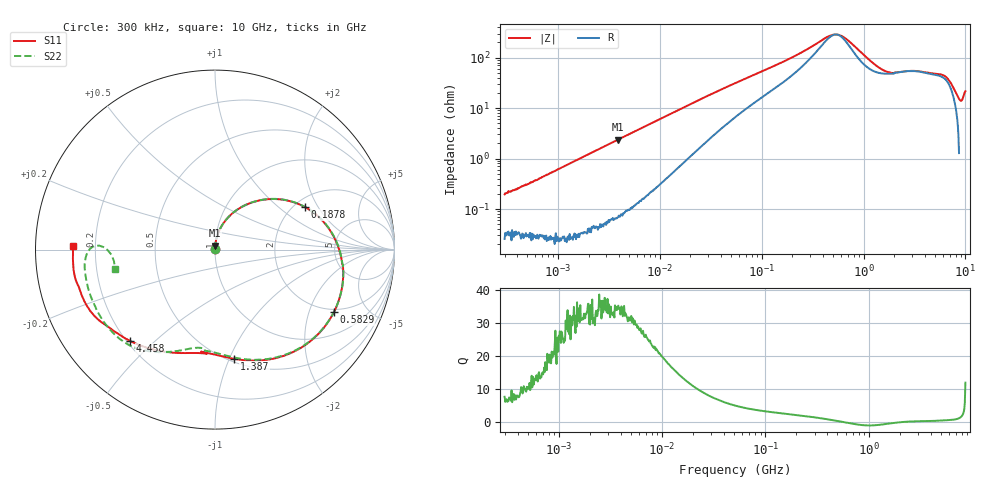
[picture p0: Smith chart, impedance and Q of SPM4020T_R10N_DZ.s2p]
! S-Parameter Data Generated by TDK Corporation
! Copyright(C) 2024 TDK Corporation.
! All Rights Reserved.
! TDK P/N: SPM4020T-R10N-DZ (SMD / SMT Inductor (Coil))
! Property: L=100nH at 100kHz
! Size(LxWxT): 4.3x4.1x2mm
! Model Type: s2p (Touchstone File Format Version 1.0)
! Frequency: DC=Yes Start=0.3MHz Stop=10000MHz 802points Log-sweep
! Model Generated on May 28, 2024
! Terms and conditions regarding TDK Simulation Models:
! 1)This simulation model is being provided solely for informational
!  purposes. Please refer to the specifications of the products in
!  terms of detailed characteristics of such products.
! 2)In no event shall TDK Corporation of any of its subsidiaries be
!  liable for any loss or damage arising, directly or indirectly,
!  from any information contained in this simulation model, including,
!  but not limited to loss or damages arising from any inaccuracies,
!  omissions or errors in connection with such information.
! 3)Any and all copyrights on this simulation model are owned by
!  TDK Corporation.  Duplication or redistribution of this simulation
!  model without prior written permission from TDK Corporation
!  is prohibited.
! 4)This simulation model is subject to any modification or change
!  without any prior notice.
! 5)Neither TDK Corporation nor any of its subsidiaries shall make any
!  warranty, express or implied, including but not limited to the
!  correctness, implied warranties of merchantability and fitness for
!  a particular purpose with respect to this simulation models.
! 6)The use of this simulation model shall be deemed to have consented
!  to the terms and conditions hereof.
! Port Assignments:
!  1 ---@@@--- 2
! Applicable Conditions:
!  Temperature = 25 degC
!  DC Bias Current = 0 A
!  Small Signal Operation
# Hz S MA R 50
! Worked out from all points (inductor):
!   801 points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, 300 kHz to 10 GHz, reference 50 ohm
!   read as one part in series: L = 100 nH near 318.3 kHz
!   highest Q = 35 at 3.867 MHz (marker M1), where L = 96.8 nH
!   self-resonance near 540.8 MHz
!   S11 on the Smith chart (normalised r, x): 300 kHz: 1.00, +0.00; 187.8 MHz: 2.26, +1.55; 582.9 MHz: 1.87, -2.96; 1.387 GHz: 0.53, -1.04; 4.458 GHz: 0.21, -0.42; 10 GHz: 0.12, +0.01
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300000  0.002422 90.5  0.9994 -0.1  0.9993 -0.1  0.002479 96.0
583966  0.003627 86.5  0.9997 -0.2  0.9996 -0.2  0.003737 87.5
1713600  0.01003 88.1  0.9995 -0.6  0.9995 -0.6  0.01008 88.5
3866967  0.0222 86.8  0.999 -1.4  0.9991 -1.4  0.02224 87.1
9671944  0.05484 83.5  0.9955 -3.5  0.9957 -3.5  0.05485 83.5
2.66222e7  0.1446 73.4  0.9713 -9.4  0.9716 -9.4  0.1446 73.4
5.477226e7  0.2646 59.7  0.9066 -17.2  0.9068 -17.2  0.2646 59.8
1.112655e8  0.4224 41.8  0.773 -28.0  0.7731 -28.0  0.4224 42.0
1.878293e8  0.5533 25.4  0.6179 -37.4  0.6179 -37.4  0.5535 25.6
3.126428e8  0.6711 5.0  0.418 -43.2  0.4181 -43.2  0.6713 5.3
4.74732e8  0.7373 -15.8  0.2653 -30.2  0.2653 -30.2  0.7371 -15.4
5.82867e8  0.7486 -27.7  0.2532 -12.6  0.2532 -12.6  0.7483 -27.3
8.872678e8  0.7133 -54.2  0.3899 0.3  0.3898 0.3  0.7116 -53.8
1.387199e9  0.6183 -80.0  0.5133 -20.6  0.5133 -20.6  0.6113 -79.8
1.767019e9  0.5817 -91.6  0.5134 -36.5  0.5134 -36.5  0.5719 -90.8
2.629198e9  0.5968 -105.1  0.438 -61.1  0.4379 -61.1  0.5718 -104.8
4.457691e9  0.6955 -133.0  0.304 -93.2  0.304 -93.2  0.6999 -127.9
6.41458e9  0.7497 -147.2  0.2284 -119.0  0.2284 -119.0  0.7344 -142.1
7.06055e9  0.7751 -154.0  0.2059 -127.9  0.2059 -127.9  0.7393 -150.4
8.211115e9  0.7867 -164.6  0.1624 -142.4  0.1625 -142.5  0.7358 -168.6
9.217363e9  0.7953 -172.9  0.1269 -152.0  0.1271 -151.9  0.6841 178.8
1e10  0.7925 178.7  0.1074 -146.9  0.1074 -146.9  0.5679 -169.0
